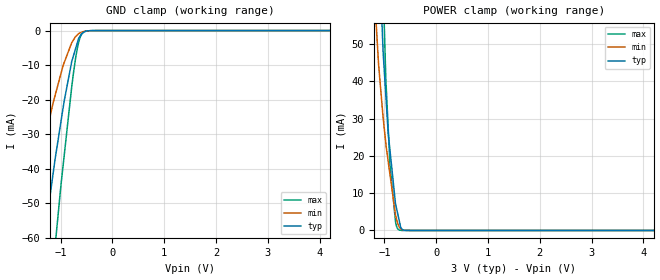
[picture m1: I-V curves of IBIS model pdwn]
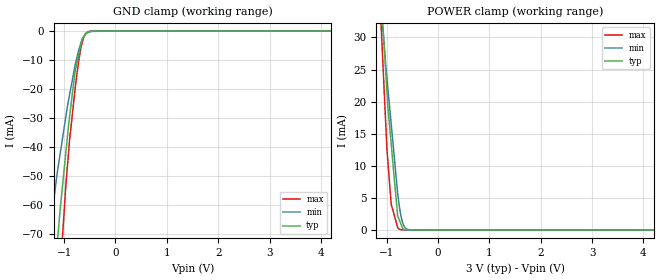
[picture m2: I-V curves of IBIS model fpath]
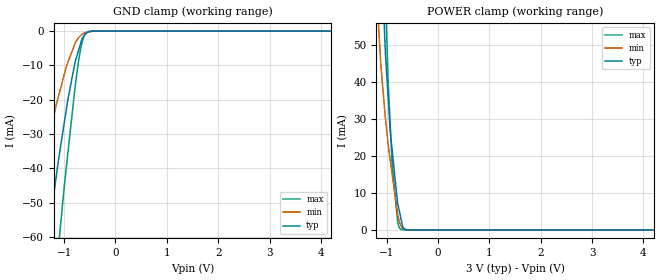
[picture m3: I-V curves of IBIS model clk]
|Texas Instruments Incorporated
| 4MSPS, 24-Bit Analog-to-Digital Converter
| Marketing part#   Digital Voltage Range   Package-type   #pins
| ADS1675IPAG   2.85V - 3.15V   TQFP   64
| ADS1675IPAGR   2.85V - 3.15V   TQFP   64
[IBIS Ver]   3.2
[File name]   ads1675.ibs
|SIMDE Ver   V3.0 - 201009 - RHL4 - Build 457
[File Rev]   1.0
[Date]   5/5/2011
[Source]
| Texas Instruments Incorporated.
| Analog-eLab Design Center, HPA
| 12500 TI Blvd
| Dallas, TX -75243
| e-mail: elab_ibis@list.ti.com
| -Model generated from simulations in TISPICE
[Notes]   Revision History:
| Rev 1.0: 5/5/2011
| - Initial version of the model
| - Model generated from simulations in TISPICE
| - Model matched to SPICE simulation
| - C_comp although listed in numerical order of value are
|   obtained from varying PVT conditions. For PVT conditions for
|   each specific value refer the buffer description under
|   respective [Model]. IBIS model user is responsible for using
|   appropriate C_comp to simulate for Signal Integrity.
|*   EXCEPTION:   *
|*   - For model dout_lvds, Rising waveform will not reach PU_ref   *
|*   and Falling waveform will not start from PU_ref. This is due to   *
|*   the fact that VT table generation is done using V_fix=Vcmt   *
[Disclaimer]
| This model is designed as an aid for customers of Texas Instruments.
| TI and its licensors and suppliers make no warranties, either expressed
| or implied, with respect to this  model, including the warranties of
| merchantability or fitness for a particular purpose. The model is
| provided solely on an "as is" basis. The entire risk as to its quality
| and performance is with the customer.
[Copyright]
 (C) Copyright 2011 Texas Instruments Incorporated.All rights reserved.
|   ADS1675
[Component]   ADS1675
[Manufacturer]   TI
[Package]   |64 TQFP -  PAG package
|   typ   min   max
R_pkg   0.06986   0.03975   0.07731
L_pkg   2.39736nH   2.07400nH   2.58915nH
C_pkg   0.49734pF   0.43727pF   0.56734pF
[Pin]  signal_name   model_name   R_pin   L_pin   C_pin
1   AVDD   POWER   0.03850   2.25009nH  0.51323pF
2   AGND   GND   0.03918   2.20428nH  0.57175pF
3   AGND   GND   0.03913   2.16131nH  0.56663pF
4   AINN   TERM   0.03975   2.14989nH  0.56734pF
5   AINP   TERM   0.04031   2.07400nH  0.52911pF
6   AGND   GND   0.04063   2.08140nH  0.51807pF
7   AVDD   POWER   0.04061   2.05510nH  0.50514pF
8   RBIAS   TERM   0.07511   2.36642nH  0.43789pF
9   AGND   GND   0.07439   2.35365nH  0.43899pF
10   AGND   GND   0.04024   2.02965nH  0.50643pF
11   AVDD   POWER   0.03982   2.06481nH  0.51238pF
12   AVDD   POWER   0.03944   2.08127nH  0.51764pF
13   VCM   TERM   0.07062   2.43569nH  0.52473pF
14   DGND   GND   0.06927   2.42047nH  0.52674pF
15   DGND   GND   0.06910   2.46139nH  0.53562pF
16   DGND   GND   0.07197   2.58783nH  0.48591pF
17   DGND   GND   0.07408   2.62551nH  0.48730pF
18   DGND   GND   0.07108   2.49859nH  0.53613pF
19   DGND   GND   0.07015   2.43931nH  0.52745pF
20   DGND   GND   0.07062   2.43947nH  0.52574pF
21   RSV2   GND   0.07168   2.36342nH  0.48418pF
22   RSV1   GND   0.07252   2.34786nH  0.47540pF
23   DVDD   POWER   0.07549   2.37810nH  0.46986pF
24   DVDD   POWER   0.04103   2.07940nH  0.46683pF
25   DGND   GND   0.04081   2.06611nH  0.47072pF
26   DGND   GND   0.04027   2.01642nH  0.50697pF
27   DVDD   POWER   0.03983   2.06889nH  0.50540pF
28   _PDWN   pdwn   0.07197   2.36848nH  0.48539pF
29   SCLK_SEL   pdwn   0.07059   2.43932nH  0.52625pF
30   _LVDS   pdwn   0.06979   2.43330nH  0.52761pF
31   DGND   GND   0.07037   2.48667nH  0.53544pF
32   LL_CONFIG   fpath   0.07199   2.58915nH  0.48510pF
33   FPATH   fpath   0.07016   2.55439nH  0.48340pF
34   DRATE[2]   fpath   0.06867   2.45320nH  0.53347pF
35   DRATE[1]   fpath   0.06926   2.41987nH  0.52524pF
36   DRATE[0]   fpath   0.07061   2.43575nH  0.52451pF
37   START   fpath   0.07177   2.36074nH  0.48460pF
38   _CS   pdwn   0.07303   2.35229nH  0.47527pF
39   OTRD   otrd   0.07617   2.38483nH  0.46932pF
40   OTRA   TERM   0.07731   2.40487nH  0.43872pF
41   _SCLK   sclk   0.07723   2.40383nH  0.43727pF
42   SCLK   sclk   0.07394   2.34560nH  0.46622pF
43   _DOUT   dout   0.07560   2.39750nH  0.47650pF
44   DOUT   dout   0.07168   2.35855nH  0.48376pF
45   _DRDY   dout   0.07317   2.47923nH  0.52642pF
46   DRDY   dout   0.06924   2.41844nH  0.52269pF
47   DGND   GND   0.06805   2.44002nH  0.53152pF
48   DVDD   POWER   0.06917   2.53177nH  0.48292pF
49   DVDD   POWER   0.03886   2.26544nH  0.51527pF
50   DGND   GND   0.03870   2.20149nH  0.56772pF
51   DGND   GND   0.03928   2.16964nH  0.56457pF
52   DVDD   POWER   0.03951   2.16393nH  0.56654pF
53   AVDD   POWER   0.03951   2.06965nH  0.52474pF
54   AGND   GND   0.03997   2.04371nH  0.51100pF
55   CLK   clk   0.07408   2.34417nH  0.46766pF
56   AGND   GND   0.07428   2.34731nH  0.43765pF
57   AGND   GND   0.04066   2.06321nH  0.46800pF
58   AVDD   POWER   0.04029   2.05717nH  0.49610pF
59   CAP1   TERM   0.07408   2.36770nH  0.47493pF
60   VREFN   TERM   0.07185   2.35823nH  0.48504pF
61   VREFN   TERM   0.07058   2.43083nH  0.52417pF
62   CAP2   TERM   0.06925   2.41539nH  0.52491pF
63   VREFP   TERM   0.06852   2.44553nH  0.53265pF
64   VREFP   TERM   0.06948   2.53628nH  0.48269pF
[Diff_pin]   inv_pin   vdiff   tdelay_typ   tdelay_min   tdelay_max
42   41   NA   0   0   0
44   43   NA   0   0   0
46   45   NA   0   0   0
|   Model Selectors
[Model Selector] dout
dout_cmos  3.0V 3-state CMOS
dout_lvds  3.0V Differential output
[Model Selector] sclk
sclk_cmos  3.0V I/O CMOS
dout_lvds  3.0V Differential output
[Model]  TERM
Model_type Terminator
C_comp   1.0e-20F  1.0e-20F  1.0e-20F
|   typ   min   max
[Voltage Range]   3.0V   2.85V   3.15V
[POWER Clamp Reference]   3.0V   2.85V   3.15V
[GND Clamp Reference]   0V   0V   0V
|Ambient Temperature   25   85   -40
|Junction Temperature
[Temperature Range]   51   111   -40
| Models and submodels in the file (8): pdwn (Input), fpath (Input), clk (Input), otrd (3-state), sclk_cmos (I/O), dout_cmos (3-state), dout_lvds (Output), TERM (Terminator)
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|   pdwn Model
[Model]   pdwn
Model_type   Input
Vinl = 0.9
Vinh = 2.1
|   typ   min   max
|   (nom PVT)   (Fast PVT)   (slow PVT)
|C_comp from frequency method(F=32MHz)
|Average
C_comp   7.392e-12   6.661e-12   7.996e-12
|C_comp from L-C Tank method(L=1nH)
|Resonant Frequency(Hz)   1.96e9   2.02e9   1.91e9
|C_comp   6.600e-12   6.214e-12   6.950e-12
| Where nom  PVT is Nominal Process,  3V,  51C
|   Fast PVT is Strong Process,   3.15V,  -40C
|   Slow PVT is Weak Process,   2.85V,  111C
[Model Spec]
Vinl   0.9   0.855   0.945
Vinh   2.1   1.995   2.205
[Voltage Range]   3   2.85   3.15
|Ambient Temperature   25   85   -40
|Junction Temperature
[Temperature Range]   51   111   -40
[Power Clamp Reference]   3   2.85   3.15
[GND Clamp Reference]   0   0   0
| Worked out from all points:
|   GND clamp passes 1 mA (typ) near -0.60 V on its own axis
|   POWER clamp passes 1 mA (typ) near -0.69 V on its own axis
[GND Clamp]
|   Voltage   I(typ)   I(min)   I(max)
-3V       -281.2mA   -190.5mA   -373.1mA
-1.87V    -129.2mA   -77.73mA   -186.5mA
-1.61V    -95.81mA   -55.14mA   -143.7mA
-1.308V   -59.14mA   -32.02mA   -93.89mA
-1.107V   -37.24mA   -18.79mA   -62.39mA
-992.2mV  -26.21mA   -12.37mA   -44.52mA
-786mV    -8.975mA   -3.525mA   -16.27mA
-708.7mV  -5.107mA   -1.725mA   -7.754mA
-641.2mV  -1.97mA    -798.7uA   -2.813mA
-557.5mV  -527.6uA   -270.9uA   -404.7uA
-384.3mV  -6.082uA   -27.05uA   -1.446uA
6V        0A         0A         0A
[POWER Clamp]
|   Voltage   I(typ)   I(min)   I(max)
-3V       1.036A     846.7mA    1.359A
-1.197V   113.3mA    64.7mA     161.7mA
-1.131V   85.4mA     49mA       123.4mA
-1.065V   62.05mA    36.83mA    84.81mA
-1.023V   47.55mA    30.11mA    64.93mA
-927mV    26.22mA    18.57mA    27.64mA
-891.4mV  21.43mA    14.97mA    17.43mA
-784.3mV  7.123mA    4.124mA    2.232mA
-711.9mV  2.53mA     948.4uA    104.4uA
-651mV    263.1uA    187.9uA    6.481uA
-519mV    2.66uA     25.44uA    1.143uA
6V        0A         0A         0A
|   fpath Model
[Model]   fpath
Model_type   Input
Vinl = 0.9
Vinh = 2.1
|   typ   min   max
|C_comp from frequency method(F=32MHz)
|Average
|C_comp   3.912e-12   3.081e-12   4.659e-12
|C_comp from L-C Tank method(L=1nH)
|Resonant Frequency(Hz)   2.88e9   3.15e9   2.65e9
C_comp   3.057e-12   2.555e-12   3.611e-12
| Where nom  PVT is Nominal Process,  3V,  51C
|   Fast PVT is Strong Process,   3.15V,  -40C
|   Slow PVT is Weak Process,   2.85V,  111C
[Model Spec]
Vinl   0.9   0.855   0.945
Vinh   2.1   1.995   2.205
[Voltage Range]   3   2.85   3.15
|Ambient Temperature   25   85   -40
|Junction Temperature
[Temperature Range]   51   111   -40
[Power Clamp Reference]   3   2.85   3.15
[GND Clamp Reference]   0   0   0
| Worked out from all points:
|   GND clamp passes 1 mA (typ) near -0.59 V on its own axis
|   POWER clamp passes 1 mA (typ) near -0.72 V on its own axis
[GND Clamp]
|   Voltage   I(typ)   I(min)   I(max)
-3V       -486.9mA   -340.5mA   -702.3mA
-1.5V     -147.1mA   -98.91mA   -215.8mA
-1.206V   -87.72mA   -58.85mA   -122.4mA
-1.129V   -71.97mA   -48.27mA   -98.96mA
-1.062V   -58.61mA   -40.5mA    -78.96mA
-963.9mV  -41.41mA   -29.2mA    -52.67mA
-909mV    -31.74mA   -23.43mA   -40.92mA
-786mV    -13.85mA   -11.73mA   -19.93mA
-711.9mV  -7.84mA    -6.358mA   -9.904mA
-652.1mV  -2.987mA   -3.104mA   -4.185mA
-513.4mV  -203uA     -353.2uA   -143.9uA
6V        0A         0A         0A
[POWER Clamp]
|   Voltage   I(typ)   I(min)   I(max)
-3V       215.5mA    189.7mA    255.8mA
-1.611V   100.9mA    86.62mA    117.9mA
-1.015V   24.4mA     25.49mA    16.15mA
-992.2mV  21.53mA    23.57mA    12.43mA
-972mV    18.94mA    21.83mA    10.35mA
-910.3mV  13.4mA     16.52mA    4.015mA
-786mV    2.246mA    5.807mA    421.3uA
-737.1mV  1.25mA     2.937mA    65.75uA
-701.1mV  517.1uA    1.506mA    39.77uA
-661.2mV  93.62uA    598.4uA    10.98uA
-561.5mV  7.79uA     37.02uA    1.406uA
6V        0A         0A         0A
|   clk Model
[Model]   clk
Model_type   Input
Vinl = 0.9
Vinh = 2.1
|   typ   min   max
|   (nom PVT)   (Fast PVT)   (slow PVT)
|C_comp from frequency method(F=32MHz)
|Average
C_comp   7.339e-12   6.608e-12   7.938e-12
|C_comp from L-C Tank method(L=1nH)
|Resonant Frequency(Hz)   1.96e9   2.02e9   1.91e9
|C_comp   6.600e-12   6.214e-12   6.950e-12
| Where nom  PVT is Nominal Process,  3V,  51C
|   Fast PVT is Strong Process,   3.15V,  -40C
|   Slow PVT is Weak Process,   2.85V,  111C
[Model Spec]
Vinl   0.9   0.855   0.945
Vinh   2.1   1.995   2.205
[Voltage Range]   3   2.85   3.15
|Ambient Temperature   25   85   -40
|Junction Temperature
[Temperature Range]   51   111   -40
[Power Clamp Reference]   3   2.85   3.15
[GND Clamp Reference]   0   0   0
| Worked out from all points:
|   GND clamp passes 1 mA (typ) near -0.60 V on its own axis
|   POWER clamp passes 1 mA (typ) near -0.69 V on its own axis
[GND Clamp]
|   Voltage   I(typ)   I(min)   I(max)
-3V       -281.4mA   -190.7mA   -373.5mA
-1.87V    -129.4mA   -77.86mA   -186.7mA
-1.61V    -95.92mA   -55.24mA   -143.8mA
-1.308V   -59.21mA   -32.08mA   -93.96mA
-1.107V   -37.28mA   -18.84mA   -62.42mA
-992.2mV  -26.24mA   -12.41mA   -44.54mA
-786mV    -8.983mA   -3.54mA    -16.28mA
-708.7mV  -5.111mA   -1.734mA   -7.757mA
-641.2mV  -1.97mA    -802.3uA   -2.814mA
-557.5mV  -527.8uA   -271.4uA   -404.7uA
-384.3mV  -6.082uA   -27.05uA   -1.446uA
6V        0A         0A         0A
[POWER Clamp]
|   Voltage   I(typ)   I(min)   I(max)
-3V       1.037A     846.9mA    1.359A
-1.197V   113.3mA    64.75mA    161.8mA
-1.131V   85.44mA    49.04mA    123.4mA
-1.065V   62.07mA    36.86mA    84.82mA
-1.023V   47.57mA    30.14mA    64.94mA
-927mV    26.23mA    18.53mA    27.64mA
-891.4mV  21.44mA    14.94mA    17.43mA
-784.3mV  7.124mA    4.13mA     2.232mA
-711.9mV  2.53mA     950.3uA    104.4uA
-651mV    263.1uA    188.2uA    6.481uA
-519mV    2.66uA     25.46uA    1.143uA
6V        0A         0A         0A
